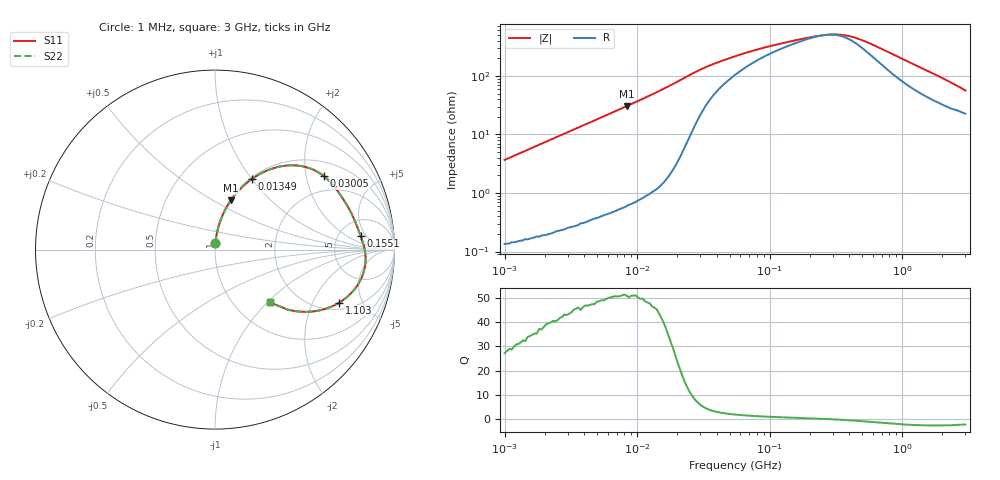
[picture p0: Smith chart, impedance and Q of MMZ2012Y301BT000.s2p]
! S-parameter Generated by TDK Corporation
! Copyright(C) 2016 TDK Corporation.
! All Rights Reserved.
! TDK P/N: MMZ2012Y301BT000 (Chip Beads)
! Property: |Z|=300¶ at 100MHz
! Size(LxWxT): 2x1.25x0.85mm, 0.079x0.049x0.033inches
! Model Type: s2p (Touchstone File Format Version 1.0)
! Frequency: DC=Yes Start=1MHz Stop=3000MHz 202points Log-sweep
! Note: This model was converted from impedance.
! Model Generated on May. 16, 2016
! Hash(MD5):
! Port Assignments:
!  1 ---@@@--- 2
! Applicable Conditions:
!  Temperature = 25 degC
!  DC Bias Current = 0 A
!  Small Signal Operation
! Terms and conditions regarding TDK Simulation Models
! (1)This simulation model is being provided solely for informational purposes. Please refer to the specifications of the products in terms of detailed characteristics of such products.
! (2)In no event shall TDK Corporation of any of its subsidiaries be liable for any loss or damage arising, directly or indirectly,
!  From any information contained in this simulation model, including, but not limited to loss or damages arising from any inaccuracies, omissions or errors in connection with such information.
! (3)Any and all copyrights on this simulation model are owned by TDK Corporation.
!  Duplication or redistribution of this simulation model without prior written permission from TDK Corporation is prohibited.
! (4)This simulation model is subject to any modification or change without any prior notice.
! (5)Neither TDK Corporation nor any of its subsidiaries shall make any warranty, express or implied,
!  Including but not limited to the correctness, implied warranties of merchantability and fitness for a particular purpose with respect to this simulation models.
! (6)The use of this simulation model shall be deemed to have consented to the terms and conditions hereof.
# MHz S MA R 50
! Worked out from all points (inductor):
!   201 points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, 1 MHz to 3 GHz, reference 50 ohm
!   read as one part in series: L = 583 nH near 1.041 MHz
!   highest Q = 51 at 8.345 MHz (marker M1), where L = 581 nH
!   self-resonance near 267.8 MHz
!   S11 on the Smith chart (normalised r, x): 1 MHz: 1.00, +0.07; 13.49 MHz: 1.02, +1.01; 30.05 MHz: 1.44, +2.53; 155.1 MHz: 8.20, +3.65; 1.103 GHz: 2.38, -3.25; 3 GHz: 1.45, -1.03
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1  0.03664 85.8  0.998 -2.1  0.998 -2.1  0.03664 85.8
2.13957  0.07774 84.1  0.995 -4.5  0.995 -4.5  0.07774 84.1
3.900413  0.1401 80.7  0.9871 -8.0  0.9871 -8.0  0.1401 80.7
8.345207  0.2899 72.0  0.9514 -16.8  0.9514 -16.8  0.2899 72.0
13.49163  0.4459 62.3  0.8855 -26.5  0.8855 -26.5  0.4459 62.3
14.61624  0.4771 60.2  0.868 -28.5  0.868 -28.5  0.4771 60.2
18.58443  0.5769 52.8  0.7975 -35.2  0.7975 -35.2  0.5769 52.8
21.81181  0.6428 46.9  0.7316 -39.9  0.7316 -39.9  0.6428 46.9
30.0453  0.7312 34.1  0.5694 -46.1  0.5694 -46.1  0.7312 34.1
38.20236  0.7549 26.4  0.4668 -46.0  0.4668 -46.0  0.7549 26.4
54.77226  0.7765 18.4  0.3592 -42.9  0.3592 -42.9  0.7765 18.4
88.54986  0.7968 11.1  0.2663 -35.1  0.2663 -35.1  0.7968 11.1
155.0909  0.8156 5.2  0.202 -21.6  0.202 -21.6  0.8156 5.2
213.6344  0.8266 2.3  0.177 -10.6  0.177 -10.6  0.8266 2.3
294.2768  0.8365 -1.0  0.1644 5.2  0.1644 5.2  0.8365 -1.0
374.1707  0.841 -3.9  0.1709 19.6  0.1709 19.6  0.841 -3.9
495.1867  0.8388 -7.9  0.2047 34.3  0.2047 34.3  0.8388 -7.9
800.5644  0.8048 -16.4  0.3224 45.0  0.3224 45.0  0.8048 -16.4
1102.76  0.7527 -23.1  0.4269 43.8  0.4269 43.8  0.7527 -23.1
1855.641  0.6098 -34.6  0.6071 34.8  0.6071 34.8  0.6098 -34.6
2359.433  0.5208 -39.8  0.6859 29.1  0.6859 29.1  0.5208 -39.8
3000  0.4229 -43.5  0.7518 22.8  0.7518 22.8  0.4229 -43.5
